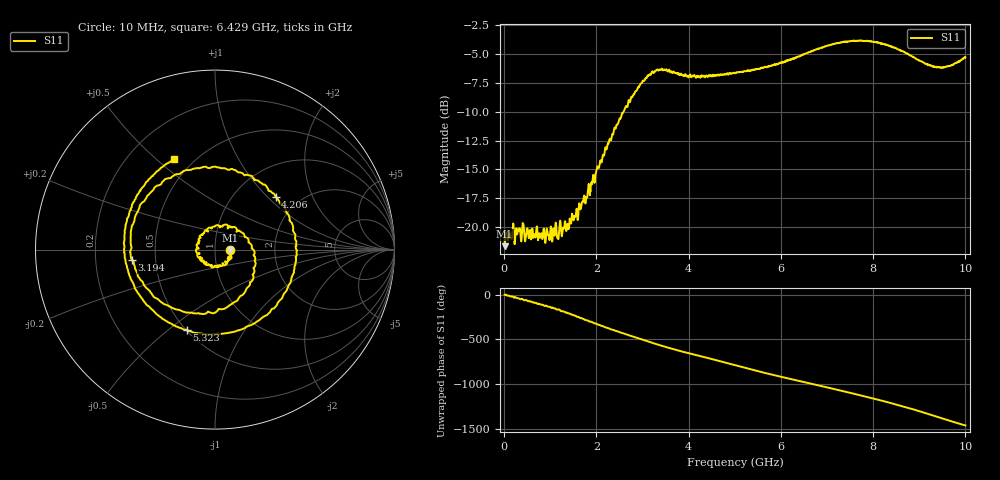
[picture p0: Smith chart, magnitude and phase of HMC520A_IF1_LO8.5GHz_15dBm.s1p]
! Analog Devices, Inc.
! 1 Analog Way
! Wilmington, MA 01887
! http://www.analog.com
! Date:  2021-09-07 NN
! Board Name:  EV1HMC520ALC4 Revision A with HMC520ALC4 installed
! File Description:  S-Parameters for evaluation board without connectors or board loss de-embedded
! File Generation:  Calibrated Network Analyzer
! Chip Part Number:  HMC520A
! Chip Description:  GaAs, MMIC, IQ Mixer
! Chip Frequency:  6 to 10 GHz
! Chip Package:  LCC, 3.9 x 3.9 x 0.9 mm
! Chip State:
!  Temperature:  25C
!  LO Frequency:  8.5GHz
!  LO Power:  15dBm
! Note:
!  Analog Devices supplies this data as a sample of measured data at the evaluation board
!  ports for this product.  Your particular data for this product may vary.
!  Analog Devices reserves the right to change this data at anytime.
!  All lines below in this file are as is from the Network Analyzer.
!Keysight Technologies,N5245A,MY49151104,A.10.65.16
!Date: Wednesday, August 04, 2021 10:52:32
!Correction: S22(Full 2 Port(1,2))
!S1P File: Measurement: S22:
# Hz S  dB  R 50
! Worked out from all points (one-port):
!   1601 points, 10 MHz to 10 GHz, reference 50 ohm
!   lowest |S11| = -21.7 dB at 10 MHz (marker M1), VSWR 1.18, Z = 59 - j0.315 ohm
!   |S11| at or under -10 dB: start of sweep to 2.588 GHz
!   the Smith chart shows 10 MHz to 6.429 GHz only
!   S11 on the Smith chart (normalised r, x): 10 MHz: 1.18, -0.01; 3.194 GHz: 0.37, -0.05; 4.206 GHz: 1.52, +1.12; 5.323 GHz: 0.50, -0.58; 6.429 GHz: 0.39, +0.57
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1e7  -21.66 -1.8
6.655938e8  -20.67 -92.1
1.25875e9  -20.59 177.2
1.926831e9  -15.55 49.0
2.239019e9  -12.88 -10.3
2.5075e9  -10.57 -59.3
2.85715e9  -8.20 -118.2
3.194312e9  -6.64 -173.0
3.419088e9  -6.26 149.3
3.75625e9  -6.69 100.1
4.2058e9  -6.98 41.1
4.592912e9  -6.82 -10.1
5.005e9  -6.67 -66.4
5.323431e9  -6.49 -109.3
5.791712e9  -6.03 -169.7
6.25375e9  -5.43 134.5
6.428575e9  -5.13 114.4
6.915588e9  -4.41 56.7
7.227775e9  -4.05 19.0
7.5025e9  -3.89 -14.8
7.845906e9  -3.88 -57.8
8.114388e9  -4.01 -92.3
8.470281e9  -4.47 -140.4
8.75125e9  -5.01 179.5
9.069681e9  -5.68 130.6
9.338162e9  -6.10 86.9
9.706544e9  -5.96 27.2
1e10  -5.30 -17.6
